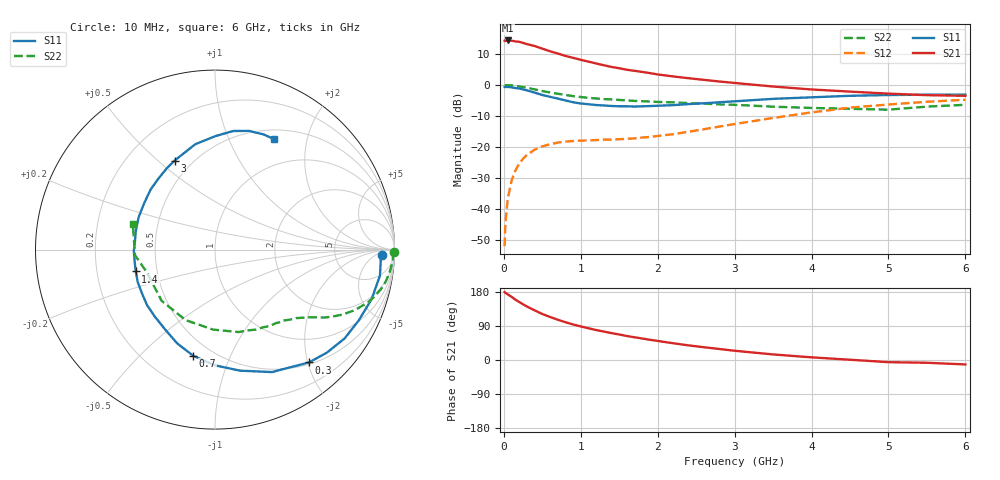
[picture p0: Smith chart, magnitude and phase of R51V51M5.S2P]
! SIEMENS Small Signal Semiconductors
! BFR183
! Si NPN RF Bipolar Junction Transistor in SOT23
! VCE = 1.5 V  IC = 1.5 mA
! Common Emitter S-Parameters:  May  1996
# GHz  S  MA  R  50
!  f  S11  S21  S12  S22
! GHz  MAG  ANG  MAG  ANG  MAG  ANG  MAG  ANG
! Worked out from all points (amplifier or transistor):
!   36 points, 10 MHz to 6 GHz, reference 50 ohm
!   highest |S21| = 14.4 dB at 50 MHz (marker M1)
!   |S21| within 3 dB of that: start of sweep to 542.1 MHz
!   unconditionally stable (mu >= 1): 1.492 GHz to 2.958 GHz
!   at 250 MHz: K = 0.19, MSG = 18.7 dB, |S12| = -23.8 dB
!   at 1.4 GHz: K = 0.96, MSG = 11.7 dB, |S12| = -17.6 dB
!   at 6 GHz: K = 0.94, MSG = 0.6 dB, |S12| = -4.8 dB
!   S11 on the Smith chart (normalised r, x): 10 MHz: 24, -10; 300 MHz: 0.53, -2.02; 700 MHz: 0.40, -0.74; 1.4 GHz: 0.38, -0.12; 3 GHz: 0.40, +0.57; 6 GHz: 0.62, +1.49
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0.01  0.9319 -1.7  5.17 179.1  0.0025 92.0  0.9969 -0.8
0.02  0.9253 -3.5  5.105 177.2  0.0059 89.7  0.9917 -1.4
0.05  0.9306 -8.9  5.229 173.3  0.0143 84.7  0.9926 -3.6
0.1  0.9152 -17.6  5.188 166.7  0.0285 80.7  0.9821 -7.1
0.15  0.8928 -26.2  5.046 159.3  0.0416 74.8  0.9687 -10.5
0.2  0.8756 -34.4  4.975 153.1  0.0538 70.4  0.9492 -13.6
0.3  0.8182 -50.2  4.566 141.1  0.0744 62.0  0.9019 -19.0
0.4  0.7528 -65.0  4.253 131.1  0.0902 55.3  0.849 -23.4
0.5  0.6889 -78.3  3.855 121.4  0.1018 49.5  0.7974 -27.0
0.6  0.6445 -90.1  3.501 113.6  0.1107 45.2  0.7563 -29.5
0.7  0.6039 -101.6  3.218 106.4  0.1173 41.9  0.722 -31.6
0.8  0.5632 -112.0  2.947 99.8  0.1217 39.2  0.6893 -33.3
0.9  0.5261 -121.5  2.74 93.8  0.1245 37.7  0.6607 -34.8
1.1  0.4888 -140.8  2.382 83.8  0.1276 35.8  0.6203 -37.7
1.4  0.458 -164.6  1.953 70.9  0.1313 36.1  0.5843 -41.5
1.8  0.4527 167.5  1.624 56.7  0.1417 41.5  0.5472 -46.9
2.2  0.4721 146.5  1.374 44.3  0.1602 47.3  0.5245 -54.1
3  0.5446 114.4  1.078 24.4  0.234 52.0  0.4781 -73.9
3.5  0.5969 100.7  0.943 14.7  0.2934 49.1  0.4461 -91.2
4.5  0.6684 81.3  0.781 0.7  0.4307 36.6  0.4122 -136.2
5.5  0.6964 67.2  0.684 -7.3  0.5356 21.3  0.4469 -176.0
6  0.698 61.7  0.668 -11.7  0.5771 11.8  0.4787 162.9
